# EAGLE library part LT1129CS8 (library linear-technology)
VOLTAGE REGULATOR with shutdown
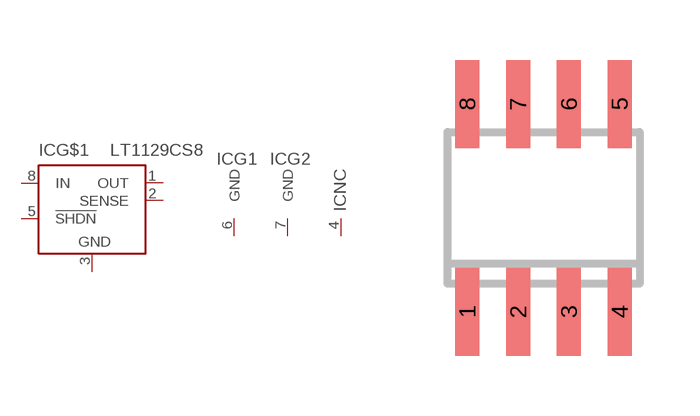
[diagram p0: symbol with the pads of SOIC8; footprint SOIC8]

Designator prefix IC; gates G$1=LT1129 G1=GND G2=GND NC=NC

## LT1129CS8 (MPN: LT1129CS8-5#PBF; OC_FARNELL: 1273576; OC_NEWARK: 57M2078)  [SOIC8]
1  G$1:OUT  out
2  G$1:SENSE  in
3  G$1:GND  pwr
4  NC:NC  nc
5  G$1:!SHDN  in
6  G1:GND  pwr
7  G2:GND  pwr
8  G$1:IN  in

## Footprint SOIC8 (pad centres in mm)
Small Outline IC
smd 0.6 x 2.2: 1 -1.905,-2.6; 2 -0.635,-2.6; 3 0.635,-2.6; 4 1.905,-2.6; 5 1.905,2.6; 6 0.635,2.6; 7 -0.635,2.6; 8 -1.905,2.6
